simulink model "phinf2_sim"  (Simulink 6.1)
settings: Solver=ode45  StartTime=0.0  StopTime=250  RelTol=1e-3
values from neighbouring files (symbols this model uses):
  A = [0 1 0 0;-P/M1 -D/M1 P/M1 0;0 0 0 1;P/M2 0 -P/M2 0]    [DED042_LQG.m]    (also in phinf2.m; podklad.m = [dh1_h10 dh1_h20 0; testx.m = [ -0.195 0.195; 0.195 -0.205]; kockaLQG.m = [0 1 0 0 0)
  B = [0;0;0;1/M2]    [DED042_LQG.m]    (also in phinf2.m; podklad.m = [dh1_q0; testx.m = [0.0047; 0]; kockaLQG.m = [0)
  B1 = [B zeros(m,1)]    [phinf2.m]    (also in testx.m = [1 0; 0 0;]; kulicka_na_tyci_reg_funkcnirobustBEZVAH_podklad.m = [7.14 0;0 0])
  B2 = B    [phinf2.m]    (also in testx.m; kulicka_na_tyci_reg_funkcnirobustBEZVAH_podklad.m = [7.14;0])
  C = [0 0 1 0]    [DED042_LQG.m]    (also in phinf2.m; podklad.m = [0 0 1]; testx.m = [0 1]; kockaLQG.m = [1 0 0 0 0])
  C1 = [C;zeros(1,m)]    [phinf2.m]    (also in testx.m = [C; 0 0]; kulicka_na_tyci_reg_funkcnirobustBEZVAH_podklad.m = [0 1;0 0])
  C2 = C    [phinf2.m]    (also in testx.m; kulicka_na_tyci_reg_funkcnirobustBEZVAH_podklad.m = [0 1])
  D = 0    [DED042_LQG.m]    (also in phinf2.m = [0]; podklad.m; testx.m = [0]; kockaLQG.m = [0])
  D11 = [0 0;0 0]    [phinf2.m]    (also in testx.m = [0 0; 0 0]; kulicka_na_tyci_reg_funkcnirobustBEZVAH_podklad.m)
  D12 = [0;1]    [phinf2.m]    (also in testx.m; kulicka_na_tyci_reg_funkcnirobustBEZVAH_podklad.m)
  D21 = [0 1]    [phinf2.m]    (also in testx.m; kulicka_na_tyci_reg_funkcnirobustBEZVAH_podklad.m)
  D22 = 0    [phinf2.m]    (also in testx.m = [0]; kulicka_na_tyci_reg_funkcnirobustBEZVAH_podklad.m)
  Ng = lqr_kompenzace(A,B,C,D,K)    [DED042_LQG.m]    (also in lqr_kompenzace.m = Nu + K*Nx; phinf2.m = -num(length(num))/den(length(den)); testx.m; kockaLQG.m)
undefined symbols (not defined in the file or in its folder): KA, KB, KC, KD

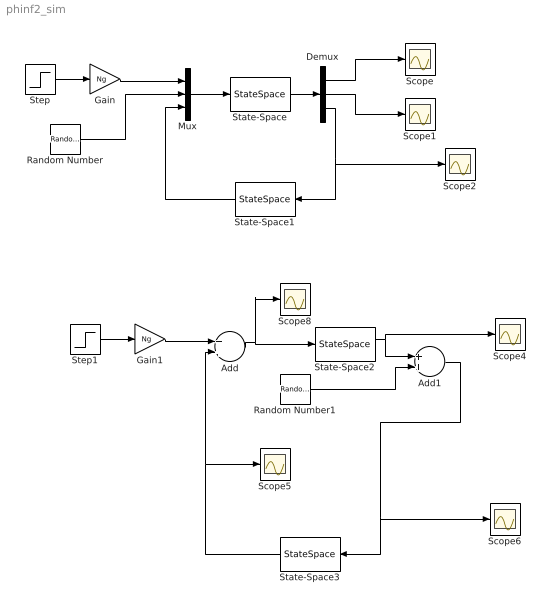
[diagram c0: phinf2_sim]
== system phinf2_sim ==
  Add : Sum  OutScaling=2^-10
  Add1 : Sum  OutScaling=2^-10
  Demux : Demux  Outputs=3
  Gain : Gain  Gain=Ng
  Gain1 : Gain  Gain=Ng
  Mux : Mux  Inputs=3
  Random Number : RandomNumber  Variance=0  SampleTime=0
  Random Number1 : RandomNumber  Variance=0  SampleTime=0
  Scope{,1..2,4..6,8} (7 alike) : Scope
  State-Space : StateSpace  A=A  B=[B1 B2]  C=[C1;C2]  D=[D11 D12;D21 D22]
  State-Space1 : StateSpace  Orientation=left  A=KA  B=KB  C=KC  D=KD
  State-Space2 : StateSpace  A=A  B=B  C=C  D=D
  State-Space3 : StateSpace  Orientation=left  A=KA  B=KB  C=KC  D=KD
  Step : Step  Time=0  SampleTime=0
  Step1 : Step  Time=0  SampleTime=0
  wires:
  Mux/1 -> State-Space/1
  State-Space/1 -> Demux/1
  Random Number/1 -> Mux/2
  State-Space1/1 -> Mux/3
  Demux/1 -> Scope/1
  Demux/2 -> Scope1/1
  Demux/3 -> Scope2/1, State-Space1/1
  Gain/1 -> Mux/1
  Step/1 -> Gain/1
  Random Number1/1 -> Add1/2
  Gain1/1 -> Add/1
  Step1/1 -> Gain1/1
  Add/1 -> State-Space2/1, Scope8/1
  State-Space2/1 -> Add1/1, Scope4/1
  Add1/1 -> Scope6/1, State-Space3/1
  State-Space3/1 -> Scope5/1, Add/2
